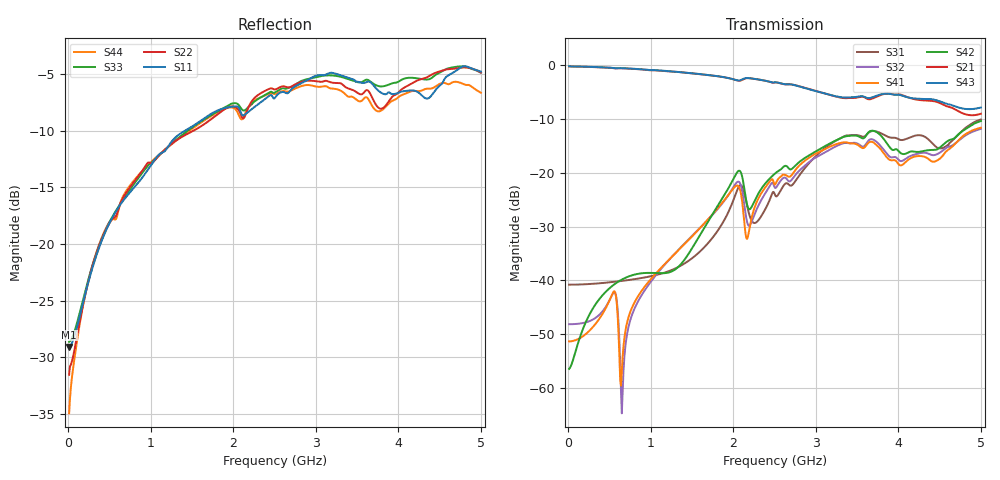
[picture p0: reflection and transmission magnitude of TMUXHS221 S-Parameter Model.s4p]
! Created Fri Aug 29 23:21:58 2025
# hz S db R 50
! 4 Port Network Data from SP1.SP block
! freq  dbS11  angS11  dbS12  angS12  dbS13  angS13  dbS14  angS14
!  dbS21  angS21  dbS22  angS22  dbS23  angS23  dbS24  angS24
!  dbS31  angS31  dbS32  angS32  dbS33  angS33  dbS34  angS34
!  dbS41  angS41  dbS42  angS42  dbS43  angS43  dbS44  angS44
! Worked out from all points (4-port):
!   1001 points, 10 MHz to 5 GHz, reference 50 ohm
!   strongest paths, dB at 10 MHz, 1.258 GHz, 2.505 GHz, 3.752 GHz, 5 GHz:
!     S43: -0.2, -1.2, -3.2, -5.6, -7.9
!     S21: -0.2, -1.2, -3.2, -5.7, -9.0
!     S42: -56.5, -38.3, -20.1, -12.6, -10.4
!     S41: -51.4, -35.6, -22.2, -15.1, -11.6
!     S32: -48.2, -35.6, -22.8, -14.5, -11.8
!     S31: -40.8, -38.1, -24.1, -12.4, -10.1
!   lowest |S11| = -29.1 dB at 10 MHz (marker M1), VSWR 1.07, Z = 53.6 - j0.263 ohm
!   |S11| at or under -10 dB: start of sweep to 1.41 GHz
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1e7  -29.10 -4.0  -0.23 -0.2  -39.92 0.6  -52.27 -2.5
     -0.23 -0.2  -31.54 54.0  -47.71 -2.4  -54.48 5.5
     -40.81 0.7  -48.17 -1.6  -28.63 -3.9  -0.24 0.2
     -51.37 -2.4  -56.48 6.9  -0.18 -0.5  -34.95 3.2
5.589e8  -17.33 -91.3  -0.56 -11.1  -40.09 33.9  -42.87 -164.9
         -0.57 -11.1  -17.65 -97.3  -48.76 -113.9  -40.66 75.8
         -40.28 38.9  -42.19 -142.8  -17.28 -90.5  -0.56 -11.3
         -42.04 -166.1  -40.74 78.2  -0.55 -11.3  -17.82 -100.6
6.5371e8  -16.28 -96.2  -0.56 -12.5  -40.12 40.6  -59.44 -39.4
          -0.57 -12.5  -16.04 -98.4  -47.95 -121.1  -39.76 77.3
          -40.10 45.6  -62.71 -122.2  -16.18 -94.7  -0.56 -12.6
          -55.47 -45.9  -39.82 79.4  -0.55 -12.6  -15.93 -99.1
8.6329e8  -14.44 -102.1  -0.74 -16.4  -40.04 57.4  -42.83 -112.2
          -0.75 -16.5  -13.86 -106.7  -44.39 -127.4  -38.71 81.8
          -39.64 60.8  -43.42 -115.8  -14.04 -101.6  -0.73 -16.7
          -42.54 -113.9  -38.75 83.7  -0.73 -16.6  -13.81 -108.8
2.06089e9  -7.90 -143.1  -2.87 -33.1  -22.75 129.1  -22.49 154.1
           -2.89 -33.2  -8.12 -141.7  -21.64 154.7  -19.69 122.2
           -22.75 129.4  -21.65 154.8  -7.68 -139.3  -2.84 -33.4
           -22.48 154.3  -19.67 122.5  -2.84 -33.5  -8.52 -144.5
2.17067e9  -8.38 -139.6  -2.39 -33.5  -26.42 95.5  -31.95 167.0
           -2.40 -33.5  -8.14 -133.8  -29.58 142.0  -26.17 101.6
           -26.43 94.5  -29.37 140.6  -7.98 -136.5  -2.38 -34.4
           -32.18 167.7  -26.15 102.4  -2.38 -34.4  -8.07 -137.0
5e9  -4.76 165.8  -9.01 -32.4  -10.06 86.0  -11.62 90.5
     -9.03 -32.6  -4.86 171.4  -11.84 91.6  -10.37 82.3
     -10.09 85.5  -11.84 91.9  -4.86 172.0  -7.88 -36.2
     -11.63 90.4  -10.37 82.5  -7.87 -36.3  -6.64 173.3
